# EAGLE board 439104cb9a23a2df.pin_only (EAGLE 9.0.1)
REV: E

Size 50.8 x 22.86 mm. Coordinates in mm from the lower left corner, seen from the top.
Outline: 2.54,0 48.26,0 arc90 50.8,2.54 50.8,20.32 arc90 48.26,22.86 2.54,22.86 arc90 0,20.32 0,13.97 0.51,13.46 0.51,9.4 0,8.89 0,2.54 arc90 2.54,0
Copper layers (1*16): Top 0.035mm / dielectric 1.5mm / Bottom 0.035mm
Design rules "adafruit *": minimum track width 8mil, minimum drill 15.5mil, track to track 9mil, track to pad 8mil, pad to pad 8mil, via to via 8mil, smd to smd 8mil, copper to edge 10mil, drill to drill 8mil, minimum pad ring 10mil, minimum via ring 8mil, stop-mask expansion 2mil, vias tented up to drill 20mil, thermal gap 10mil
Net classes: 1 power: width 0.305 mm; 2 gnd: width 0.254 mm
Holes 2.54 mm at 48.26,20.32 48.26,2.54

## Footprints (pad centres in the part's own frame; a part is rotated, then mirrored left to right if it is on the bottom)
0603-NO = smd 1.075 x 1: 1 -0.85,0; 2 0.85,0
0805-NO = smd 1.24 x 1.5: 1 -0.95,0; 2 0.95,0
CHIPLED_0805_NOOUTLINE = smd 1.2 x 1.2: A 0,-1.05; C 0,1.05
SOD-123 = smd 1.4 x 1.4: A 1.85,0; C -1.85,0
B1,27 = smd 1.27 x 1.27: TP 0,0
1X16_ROUND = drill 1 pad 1.676: 1 -19.05,0; 2 -16.51,0; 3 -13.97,0; 4 -11.43,0; 5 -8.89,0; 6 -6.35,0; 7 -3.81,0; 8 -1.27,0; 9 1.27,0; 10 3.81,0; 11 6.35,0; 12 8.89,0; 13 11.43,0; 14 13.97,0; 15 16.51,0; 16 19.05,0
1X12_ROUND = drill 1 pad 1.676: 1 -13.97,0; 2 -11.43,0; 3 -8.89,0; 4 -6.35,0; 5 -3.81,0; 6 -1.27,0; 7 1.27,0; 8 3.81,0; 9 6.35,0; 10 8.89,0; 11 11.43,0; 12 13.97,0
INDUCTOR_1007 = smd 1.016 x 2.2: P$1 -1.127,0; P$2 1.127,0
LED3535 = smd 1 x 0.85: 1 -1.75,0.875; 2 -1.75,-0.875; 3 1.75,-0.875; 4 1.75,0.875
SOT23-R = smd 0.635 x 1.016: 1 -0.95,-1; 2 0.95,-1; 3 0,1
RESPACK_4X0603_NO = smd 0.45 x 0.9: 1 -1.3,-0.85; 2 -0.4,-0.85; 3 0.4,-0.85; 4 1.3,-0.85; 5 1.3,0.85; 6 0.4,0.85; 7 -0.4,0.85; 8 -1.3,0.85
SOLDERJUMPER_CLOSEDWIRE = smd 1.168 x 1.6: 1 -0.762,0; 2 0.762,0 | smd 0.635 x 0.203: WIRE 0,0
BTN_KMR2_4.6X2.8 = smd 0.9 x 0.9: A 2.05,0.8; A' -2.05,0.8; B 2.05,-0.8; B' -2.05,-0.8
TESTPOINT_ROUND_1.5MM = smd 1.5 x 1.5: P$1 0,0
USON8 = smd 0.5 x 0.275: 1 -1.2,0.75; 2 -1.2,0.25; 3 -1.2,-0.25; 4 -1.2,-0.75; 5 1.2,-0.75; 6 1.2,-0.25; 7 1.2,0.25; 8 1.2,0.75
SOT23-5 = smd 0.55 x 1.2: 1 -0.95,-1.3; 2 0,-1.3; 3 0.95,-1.3; 4 0.95,1.3; 5 -0.95,1.3
PQFN64-1 = smd 0.7 x 0.22: 1 -4.45,3.75; 2 -4.45,3.25; 3 -4.45,2.75; 4 -4.45,2.25; 5 -4.45,1.75; 6 -4.45,1.25; 7 -4.45,0.75; 8 -4.45,0.25; 9 -4.45,-0.25; 10 -4.45,-0.75; 11 -4.45,-1.25; 12 -4.45,-1.75; 13 -4.45,-2.25; 14 -4.45,-2.75; 15 -4.45,-3.25; 16 -4.45,-3.75; 33 4.45,-3.75; 34 4.45,-3.25; 35 4.45,-2.75; 36 4.45,-2.25; 37 4.45,-1.75; 38 4.45,-1.25; 39 4.45,-0.75; 40 4.45,-0.25; 41 4.45,0.25; 42 4.45,0.75; 43 4.45,1.25; 44 4.45,1.75; 45 4.45,2.25; 46 4.45,2.75; 47 4.45,3.25; 48 4.45,3.75 | smd 0.22 x 0.7: 17 -3.75,-4.45; 18 -3.25,-4.45; 19 -2.75,-4.45; 20 -2.25,-4.45; 21 -1.75,-4.45; 22 -1.25,-4.45; 23 -0.75,-4.45; 24 -0.25,-4.45; 25 0.25,-4.45; 26 0.75,-4.45; 27 1.25,-4.45; 28 1.75,-4.45; 29 2.25,-4.45; 30 2.75,-4.45; 31 3.25,-4.45; 32 3.75,-4.45; 49 3.75,4.45; 50 3.25,4.45; 51 2.75,4.45; 52 2.25,4.45; 53 1.75,4.45; 54 1.25,4.45; 55 0.75,4.45; 56 0.25,4.45; 57 -0.25,4.45; 58 -0.75,4.45; 59 -1.25,4.45; 60 -1.75,4.45; 61 -2.25,4.45; 62 -2.75,4.45; 63 -3.25,4.45; 64 -3.75,4.45 | smd 4.7 x 4.7: EXP 0,0
MOUNTINGHOLE_2.5_PLATED = drill 2.5 pad 3.2: P$1 0,0
FIDUCIAL_1MM = smd 1 x 1: 1 0,0
JSTPH2 = smd 1 x 4.6: 1 -1,-3.7; 2 1,-3.7 | smd 1.6 x 3.4: NC1 -3.4,1.5; NC2 3.4,1.5
XTAL3215 = smd 1.1 x 1.9: P$1 1.2,0; P$2 -1.2,0
4UCONN_20329_V2 = smd 1 x 2: BASE@1 -0.75,-2; BASE@2 0.75,-2 | smd 0.4 x 1.35: D+ 0,0.775; D- -0.65,0.775; GND 1.3,0.775; ID 0.65,0.775; VBUS -1.3,0.775 | drill 0.8 pad 1.143 offset: SPRT@1 -3.3,0.9; SPRT@2 3.3,0.9 | drill 0.9 pad 2.413 square: SPRT@3 -3.6,-1.9; SPRT@4 3.6,-1.9 | hole 0.7: -1.95,0; 1.95,0

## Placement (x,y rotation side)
C2  22pF  [0603-NO]  19.2,5.07 90 top
C3  10µF  [0805-NO]  15.75,17.27 270 top
C4  22pF  [0603-NO]  21.53,6.35 180 top
C5  10uF  [0805-NO]  35.06,18.67 0 top
C6  10µF  [0805-NO]  12.04,9.84 270 top
C7  1uF  [0603-NO]  24.91,17.78 90 top
C8  10µF  [0805-NO]  14.73,13.86 0 top
C10  1uF  [0603-NO]  29.66,5.26 180 top
C11  1uF  [0603-NO]  19.13,8.06 90 top
C12  1uF  [0603-NO]  13.86,6.5 270 top
C13  10uF  [0805-NO]  18.8,11.3 270 top
C14  1uF  [0603-NO]  11.99,4.22 0 top
C15  1uF  [0603-NO]  22.23,14.41 180 top
CHG  ORANGE  [CHIPLED_0805_NOOUTLINE]  2.41,5.59 270 top
D4  MBR120  [SOD-123]  10.35,12.32 180 top
D+  TPB1,27  [B1,27]  5.33,10.41 0 bottom
D-  TPB1,27  [B1,27]  5.33,12.45 0 bottom
JP1  [1X16_ROUND]  25.4,1.27 180 top
JP3  [1X12_ROUND]  30.48,21.59 0 top
L  RED  [CHIPLED_0805_NOOUTLINE]  2.65,17.36 90 top
L2  10uH  [INDUCTOR_1007]  21.08,11.81 270 top
LED1  WS2812B3535  [LED3535]  16.48,6.11 270 top
Q3  DMG341  [SOT23-R]  9.4,9.84 0 top
R2  1K  [0603-NO]  5.83,4.25 0 top
R3  10K  [0603-NO]  17.14,10.92 90 top
R4  10K  [0603-NO]  8.89,4.25 180 top
R5  10K  [0603-NO]  36.12,4.65 180 top
R6  10K  [0603-NO]  21.4,8.06 0 top
R7  2.2K  [0603-NO]  5.71,20.95 270 top
R8  10K\  [0603-NO]  18.41,17.97 0 top
R9  100K  [RESPACK_4X0603_NO]  22.67,17.21 90 top
SJ1  [SOLDERJUMPER_CLOSEDWIRE]  10.35,3.11 0 bottom
SW1  KMR2  [BTN_KMR2_4.6X2.8]  9.4,6.54 180 top
TP1  [TESTPOINT_ROUND_1.5MM]  18.54,5.21 0 bottom
TP2  [TESTPOINT_ROUND_1.5MM]  20.89,5.27 0 bottom
U1  2MB Flash  [USON8]  36.51,8.43 90 top
U2  AP2112-3.3  [SOT23-5]  14.73,10.92 0 top
U3  MCP73831T-2ACI/OT  [SOT23-5]  18.35,15.11 0 top
U$5  [FEATHERM4_BOT]  50.8,0 0 bottom
U$6  [FEATHERM4_TOP]  0,0 0 top
U$13  [PCBFEAT-REV-040]  1.27,17.53 0 bottom
U$14  ATSAMD51J  [PQFN64-1]  30.16,11.05 90 top
U$31  MOUNTINGHOLE2.5  [MOUNTINGHOLE_2.5_PLATED]  2.54,20.32 270 top
U$32  MOUNTINGHOLE2.5  [MOUNTINGHOLE_2.5_PLATED]  2.54,2.54 270 top
U$34  FIDUCIAL_1MM  [FIDUCIAL_1MM]  10.79,20.45 270 top
U$35  FIDUCIAL_1MM  [FIDUCIAL_1MM]  46.4,0.77 270 top
X1  JSTPH  [JSTPH2]  10.79,19.3 0 top
X2  32.768  [XTAL3215]  21.81,4.5 180 top
X3  microUSB  [4UCONN_20329_V2]  4.45,11.43 270 top

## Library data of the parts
C2-C7 C10-C15 CHG D4 JP1 JP3 L L2 LED1 Q3 R2-R9 SJ1 SW1 TP1 TP2 U1-U3 U$13 U$14 X1 X3 = microbuilder
C8 = microbuilder; COMPANY: ADAFRUIT INDUSTRIES; DRAWN: KTOWN; REV: A
D+ D- = testpad
U$5 U$6 = silks
U$31 U$32 U$34 U$35 = microbuilder; BOM: EXCLUDE
X2 = adafruit2

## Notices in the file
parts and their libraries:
microbuilder: This work is placed in the public domain, and may be freely used for commercial and non-commercial work with the following conditions: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
